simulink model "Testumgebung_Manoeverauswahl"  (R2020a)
settings: Solver=ode4  StartTime=0.0  StopTime=30.0  FixedStep=0.01  RelTol=1e-3
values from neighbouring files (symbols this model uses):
  c = [0;0]    [Testskript_Manoeverauswahl.m]

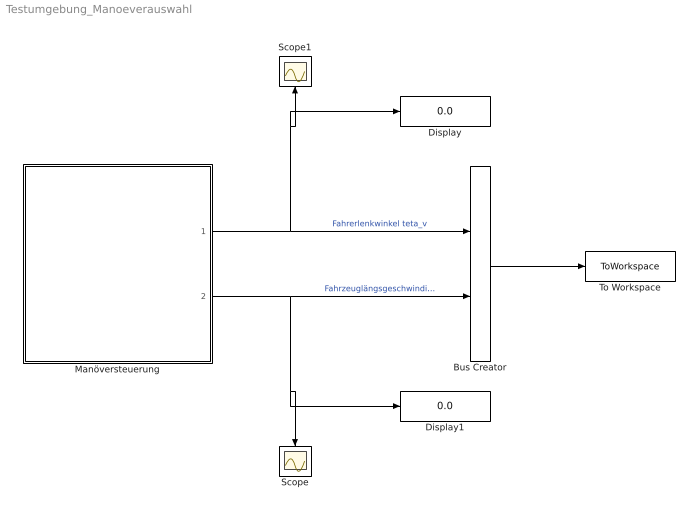
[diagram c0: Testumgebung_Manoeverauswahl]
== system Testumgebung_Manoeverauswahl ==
  Bus Creator : BusCreator  Inputs=2
  Display : Display
  Display1 : Display
  Manöversteuerung : Subsystem
  Scope : Scope
  Scope1 : Scope
  To Workspace : ToWorkspace  VariableName=simout  SaveFormat=Timeseries  SampleTime=-1
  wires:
  Manöversteuerung/2(Fahrzeuglängsgeschwindigkeit KvCx) -> Display1/1, Scope/1, Bus Creator/2  "Fahrzeuglängsgeschwindigkeit KvCx"
  Manöversteuerung/1(Fahrerlenkwinkel teta_v) -> Display/1, Scope1/1, Bus Creator/1  "Fahrerlenkwinkel teta_v"
  Bus Creator/1 -> To Workspace/1

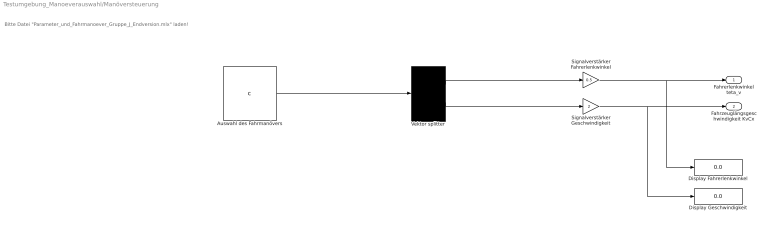
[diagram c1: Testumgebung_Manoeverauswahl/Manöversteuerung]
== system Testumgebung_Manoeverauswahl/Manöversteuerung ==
  note: Bitte Datei "Parameter_und_Fahrmanoever_Gruppe_J_Endversion.mlx" laden!
  Auswahl des Fahrmanövers : Constant  Value=c
  Display Fahrerlenkwinkel : Display
  Display Geschwindigkeit : Display
  Signalverstärker Fahrerlenkwinkel : Gain  Gain=0.5
  Signalverstärker Geschwindigkeit : Gain  Gain=2
  Vektor splitter : Demux  Outputs=2
  Fahrerlenkwinkel teta_v : Outport
  Fahrzeuglängsgeschwindigkeit KvCx : Outport  Port=2
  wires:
  Vektor splitter/1 -> Signalverstärker Fahrerlenkwinkel/1
  Vektor splitter/2 -> Signalverstärker Geschwindigkeit/1
  Signalverstärker Geschwindigkeit/1 -> Fahrzeuglängsgeschwindigkeit KvCx/1, Display Geschwindigkeit/1
  Signalverstärker Fahrerlenkwinkel/1 -> Fahrerlenkwinkel teta_v/1, Display Fahrerlenkwinkel/1
  Auswahl des Fahrmanövers/1 -> Vektor splitter/1
